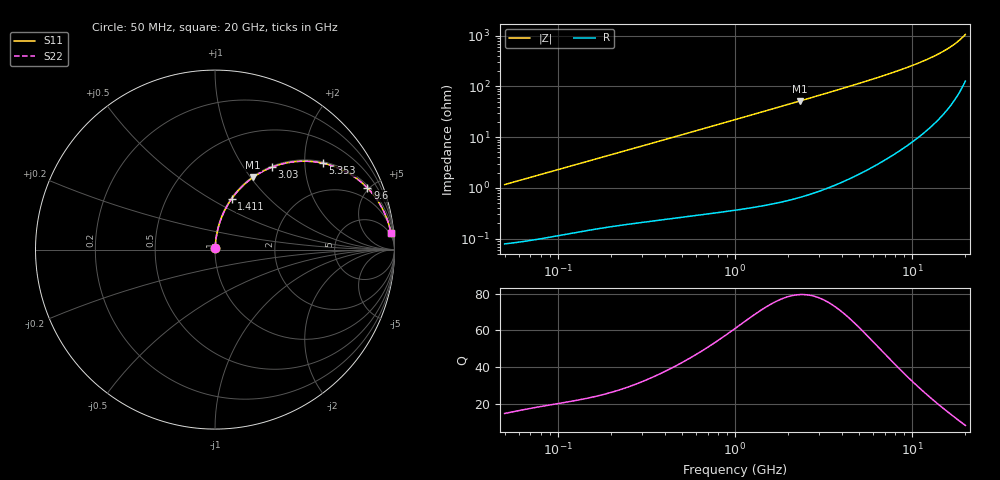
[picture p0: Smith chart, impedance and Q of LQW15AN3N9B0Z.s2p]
!Murata Part Number: LQW15AN3N9B0Z
!These Parameters are Measured in Series Mode Connection
!  o--[Z]--o
!Port1  Port2
!  o-------o
!Freq. Start=50[MHz] Stop=20[GHz], 401[Steps]
# Hz S RI R 50
!Freq.(Hz) S11(Real) S11(Imag) S21(Real) S21(Imag) S12(Real) S12(Imag) S22(Real) S22(Imag)
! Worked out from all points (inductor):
!   401 points, 50 MHz to 20 GHz, reference 50 ohm
!   read as one part in series: L = 3.68 nH near 51.52 MHz
!   highest Q = 79.5 at 2.314 GHz (marker M1), where L = 3.54 nH
!   S11 on the Smith chart (normalised r, x): 50 MHz: 1.00, +0.02; 1.411 GHz: 1.01, +0.62; 3.03 GHz: 1.02, +1.35; 5.353 GHz: 1.04, +2.46; 9.6 GHz: 1.14, +4.89; 20 GHz: 4, +21
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5e7  0.000921 0.0116  0.9991 -0.0116  0.9991 -0.0116  0.000921 0.0116
1.364002e8  0.00234 0.0309  0.9977 -0.0309  0.9977 -0.0309  0.00234 0.0309
2.33884e8  0.0046 0.0523  0.9954 -0.0523  0.9954 -0.0523  0.0046 0.0523
3.721004e8  0.00911 0.0821  0.9909 -0.0821  0.9909 -0.0821  0.00911 0.0821
6.285508e8  0.0218 0.1361  0.9782 -0.1361  0.9782 -0.1361  0.0218 0.1361
1e9  0.0499 0.2096  0.9501 -0.2096  0.9501 -0.2096  0.0499 0.2096
1.411297e9  0.0922 0.2824  0.9078 -0.2824  0.9078 -0.2824  0.0922 0.2824
1.820564e9  0.1432 0.3439  0.8568 -0.3439  0.8568 -0.3439  0.1432 0.3439
2.313601e9  0.2119 0.4024  0.7881 -0.4024  0.7881 -0.4024  0.2119 0.4024
2.728004e9  0.2723 0.4389  0.7277 -0.4389  0.7277 -0.4389  0.2723 0.4389
3.029571e9  0.3163 0.4586  0.6837 -0.4586  0.6837 -0.4586  0.3163 0.4586
3.519108e9  0.3855 0.48  0.6145 -0.48  0.6145 -0.48  0.3855 0.48
4.087748e9  0.4606 0.4913  0.5394 -0.4913  0.5394 -0.4913  0.4606 0.4913
5.352748e9  0.6006 0.4814  0.3994 -0.4814  0.3994 -0.4814  0.6006 0.4814
6.311513e9  0.6822 0.4561  0.3178 -0.4561  0.3178 -0.4561  0.6822 0.4561
7.442007e9  0.7559 0.4185  0.2441 -0.4185  0.2441 -0.4185  0.7559 0.4185
9.600142e9  0.8494 0.3433  0.1506 -0.3433  0.1506 -0.3433  0.8494 0.3433
1.220001e10  0.9129 0.2625  0.0871 -0.2625  0.0871 -0.2625  0.9129 0.2625
1.482269e10  0.9486 0.1947  0.0514 -0.1947  0.0514 -0.1947  0.9486 0.1947
1.721783e10  0.9676 0.1426  0.0324 -0.1426  0.0324 -0.1426  0.9676 0.1426
1.940974e10  0.9782 0.1012  0.0218 -0.1012  0.0218 -0.1012  0.9782 0.1012
2e10  0.9803 0.0909  0.0197 -0.0909  0.0197 -0.0909  0.9803 0.0909
